|Texas Instruments Incorporated
| MULTI-CHANNEL HIGH SPEED ADC WITH JESD204B INTERFACE
| part#   Digital Voltage Range   Package-type   #pins
| AFE58JD32   1.7V - 1.9V   BGA   289
[IBIS Ver]   4.1
[File name]   afe58jd32.ibs
[File Rev]   1.1
[Date]   9/16/2017
[Source]
| Texas Instruments Incorporated.
| Analog-eLab Design Center, HPA
| 12500 TI Blvd
| Dallas, TX -75243
[Notes]   Revision History:
| Rev 1.0: 7/01/2017
| - Initial version of the model
| - Model generated from simulations in TISPICE
| - C_comp although listed in numerical order of value are
|   obtained from varying PVT conditions. For PVT conditions for
|   each specific value refer the buffer description under
|   respective [Model]. IBIS model user is responsible for using
|   appropriate C_comp to simulate for Signal Integrity.
[Disclaimer]
| This model is designed as an aid for customers of Texas Instruments.
| TI and its licensors and suppliers make no warranties, either expressed
| or implied, with respect to this  model, including the warranties of
| merchantability or fitness for a particular purpose. The model is
| provided solely on an "as is" basis. The entire risk as to its quality
| and performance is with the customer.
[Copyright]
 (C) Copyright 2014 Texas Instruments Incorporated.All rights reserved.
|   Device
[Component]   AFE58JD32
[Manufacturer]   TI
[Package]
|   typ   min   max
R_pkg  1.000E-02   0.800E-02   1.200E-02
L_pkg  1.602E-09   1.280E-09   1.920E-09
C_pkg  0.700E-13   0.560E-13   0.840E-12
[Pin]  signal_name   model_name   R_pin   L_pin   C_pin
A1   INP31   NC   NA   NA   NA
A2   INP29   NC   NA   NA   NA
A3   INP27   NC   NA   NA   NA
A4   INP25   NC   NA   NA   NA
A5   INP23   NC   NA   NA   NA
A6   INP21   NC   NA   NA   NA
A7   INP19   NC   NA   NA   NA
A8   INP17   NC   NA   NA   NA
A9   BIAS_2P5o   NC   NA   NA   NA
A10   INP15   NC   NA   NA   NA
A11   INP13   NC   NA   NA   NA
A12   INP11   NC   NA   NA   NA
A13   INP9   NC   NA   NA   NA
A14   INP7   NC   NA   NA   NA
A15   INP5   NC   NA   NA   NA
A16   INP3   NC   NA   NA   NA
A17   INP1   NC   NA   NA   NA
B1   INM31   NC   NA   NA   NA
B2   INM29   NC   NA   NA   NA
B3   INM27   NC   NA   NA   NA
B4   INM25   NC   NA   NA   NA
B5   INM23   NC   NA   NA   NA
B6   INM21   NC   NA   NA   NA
B7   INM19   NC   NA   NA   NA
B8   INM17   NC   NA   NA   NA
B9   NC   NC   NA   NA   NA
B10   INM15   NC   NA   NA   NA
B11   INM13   NC   NA   NA   NA
B12   INM11   NC   NA   NA   NA
B13   INM9   NC   NA   NA   NA
B14   INM7   NC   NA   NA   NA
B15   INM5   NC   NA   NA   NA
B16   INM3   NC   NA   NA   NA
B17   INM1   NC   NA   NA   NA
C1   INP32   NC   NA   NA   NA
C2   INP30   NC   NA   NA   NA
C3   INP28   NC   NA   NA   NA
C4   INP26   NC   NA   NA   NA
C5   INP24   NC   NA   NA   NA
C6   INP22   NC   NA   NA   NA
C7   INP20   NC   NA   NA   NA
C8   INP18   NC   NA   NA   NA
C9   NC   NC   NA   NA   NA
C10   INP16   NC   NA   NA   NA
C11   INP14   NC   NA   NA   NA
C12   INP12   NC   NA   NA   NA
C13   INP10   NC   NA   NA   NA
C14   INP8   NC   NA   NA   NA
C15   INP6   NC   NA   NA   NA
C16   INP4   NC   NA   NA   NA
C17   INP2   NC   NA   NA   NA
D1   INM32   NC   NA   NA   NA
D2   INM30   NC   NA   NA   NA
D3   INM28   NC   NA   NA   NA
D4   INM26   NC   NA   NA   NA
D5   INM24   NC   NA   NA   NA
D6   INM22   NC   NA   NA   NA
D7   INM20   NC   NA   NA   NA
D8   INM18   NC   NA   NA   NA
D9   BIAS_2P5e   NC   NA   NA   NA
D10   INM16   NC   NA   NA   NA
D11   INM14   NC   NA   NA   NA
D12   INM12   NC   NA   NA   NA
D13   INM10   NC   NA   NA   NA
D14   INM8   NC   NA   NA   NA
D15   INM6   NC   NA   NA   NA
D16   INM4   NC   NA   NA   NA
D17   INM2   NC   NA   NA   NA
E1   AVSS   GND   NA   NA   NA
E2   AVSS   GND   NA   NA   NA
E3   AVSS		GND   NA   NA   NA
E4   LNA_IN_CMe	NC   NA   NA   NA
E5   LNA_IN_CMo   NC   NA   NA   NA
E6   AVDD_3P15   POWER   NA   NA   NA
E7   AVDD_3P15   POWER   NA   NA   NA
E8   NC   NC   NA   NA   NA
E9   NC   NC   NA   NA   NA
E10   AVDD_3P15   POWER   NA   NA   NA
E11   AVDD_3P15   POWER   NA   NA   NA
E12   AVDD_3P15   POWER   NA   NA   NA
E13   SRC_BIASo   NC   NA   NA   NA
E14   SRC_BIASe   NC   NA   NA   NA
E15   AVSS   GND   NA   NA   NA
E16   AVSS   GND   NA   NA   NA
E17   AVSS   GND   NA   NA   NA
F1   CW_OUTP_IP   NC   NA   NA   NA
F2   CW_OUTM_IP   NC   NA   NA   NA
F3   AVSS   GND   NA   NA   NA
F4   NC   NC   NA   NA   NA
F5   NC   NC   NA   NA   NA
F6   AVDD_1P9   POWER   NA   NA   NA
F7   AVDD_1P9   POWER   NA   NA   NA
F8   AVSS   GND   NA   NA   NA
F9   AVSS   GND   NA   NA   NA
F10   AVSS   GND   NA   NA   NA
F11   AVDD_1P9   POWER   NA   NA   NA
F12   AVDD_1P9   POWER   NA   NA   NA
F13   NC   NC   NA   NA   NA
F14   NC   NC   NA   NA   NA
F15   AVSS   GND   NA   NA   NA
F16   CLKP_16X   CLK_INPUT   NA   NA   NA
F17   CLKM_16X   CLK_INPUT   NA   NA   NA
G1   CW_OUTP_QP   NC   NA   NA   NA
G2   CW_OUTM_QP   NC   NA   NA   NA
G3   AVSS   GND   NA   NA   NA
G4   BAND_GAPe   NC   NA   NA   NA
G5   BAND_GAPo   NC   NA   NA   NA
G6   AVDD_1P9   POWER   NA   NA   NA
G7   AVDD_1P9   POWER   NA   NA   NA
G8   AVSS   GND   NA   NA   NA
G9   AVSS   GND   NA   NA   NA
G10   AVSS   GND   NA   NA   NA
G11   AVDD_1P9   POWER   NA   NA   NA
G12   AVDD_1P9   POWER   NA   NA   NA
G13   NC   NC   NA   NA   NA
G14   NC   NC   NA   NA   NA
G15   AVSS   GND   NA   NA   NA
G16   AVSS   GND   NA   NA   NA
G17   AVSS   GND   NA   NA   NA
H1   AVSS   GND   NA   NA   NA
H2   AVSS   GND   NA   NA   NA
H3   AVSS   GND   NA   NA   NA
H4   TGC_SLOPE   NC   NA   NA   NA
H5   TGC_PROF2   NC   NA   NA   NA
H6   AVDD_1P9   POWER   NA   NA   NA
H7   AVDD_1P9   POWER   NA   NA   NA
H8   AVSS   GND   NA   NA   NA
H9   AVSS   GND   NA   NA   NA
H10   AVSS   GND   NA   NA   NA
H11   AVDD_1P9   POWER   NA   NA   NA
H12   AVDD_1P9   POWER   NA   NA   NA
H13   AVDD_1P9   POWER   NA   NA   NA
H14   TR_EN2   NC   NA   NA   NA
H15   TR_EN3   NC   NA   NA   NA
H16   CLKM_1X   CLK_INPUT   NA   NA   NA
H17   CLKP_1X   CLK_INPUT   NA   NA   NA
J1   ADC_CLKP   CLK_INPUT   NA   NA   NA
J2   ADC_CLKM   CLK_INPUT   NA   NA   NA
J3   AVSS   GND   NA   NA   NA
J4   TGC_UP_DN   NC   NA   NA   NA
J5   TGC_PROF1   NC   NA   NA   NA
J6   AVDD_1P9   POWER   NA   NA   NA
J7   AVDD_1P9   POWER   NA   NA   NA
J8   AVSS   GND   NA   NA   NA
J9   AVSS   GND   NA   NA   NA
J10   AVSS   GND   NA   NA   NA
J11   AVDD_1P9   POWER   NA   NA   NA
J12   AVDD_1P9   POWER   NA   NA   NA
J13   NC   NC   NA   NA   NA
J14   TR_EN1   NC   NA   NA   NA
J15   TR_EN4   NC   NA   NA   NA
J16   SDOUT   SDOUT   NA   NA   NA
J17   SCLK   SCLK_INPUT   NA   NA   NA
K1   AVSS   GND   NA   NA   NA
K2   AVSS   GND   NA   NA   NA
K3   AVSS   GND   NA   NA   NA
K4   NC   NC   NA   NA   NA
K5   NC   NC   NA   NA   NA
K6   AVDD_1P8   POWER   NA   NA   NA
K7   AVDD_1P8   POWER   NA   NA   NA
K8   AVSS   GND   NA   NA   NA
K9   AVSS   GND   NA   NA   NA
K10   AVSS   GND   NA   NA   NA
K11   AVDD_1P8   POWER   NA   NA   NA
K12   AVDD_1P8   POWER   NA   NA   NA
K13   NC   NC   NA   NA   NA
K14   NC   NC   NA   NA   NA
K15   SENo   SEN   NA   NA   NA
K16   SPI_DIG_EN   SEN   NA   NA   NA
K17   SENe   SEN   NA   NA   NA
L1   SYNCP_SERDES   SYNC_INPUT   NA   NA   NA
L2   SYNCM_SERDES   SYNC_INPUT   NA   NA   NA
L3   DVDD_1P2   POWER   NA   NA   NA
L4   NC   NC   NA   NA   NA
L5   NC   NC   NA   NA   NA
L6   AVDD_1P8   POWER   NA   NA   NA
L7   AVDD_1P8   POWER   NA   NA   NA
L8   AVSS   GND   NA   NA   NA
L9   AVSS   GND   NA   NA   NA
L10   AVSS   GND   NA   NA   NA
L11   AVDD_1P8   POWER   NA   NA   NA
L12   AVDD_1P8   POWER   NA   NA   NA
L13   NC   NC   NA   NA   NA
L14   NC   NC   NA   NA   NA
L15   NC   NC   NA   NA   NA
L16   SDIN   SCLK_INPUT   NA   NA   NA
L17   RESET   SCLK_INPUT   NA   NA   NA
M1   SYSREFP_SERDES   SYNC_INPUT   NA   NA   NA
M2   SYSREFM_SERDES   SYNC_INPUT   NA   NA   NA
M3   DVSS   GND   NA   NA   NA
M4   DVDD_1P2   POWER   NA   NA   NA
M5   DVDD_1P2   POWER   NA   NA   NA
M6   DVDD_1P2   POWER   NA   NA   NA
M7   DVSS   GND   NA   NA   NA
M8   DVSS   GND   NA   NA   NA
M9   DVSS   GND   NA   NA   NA
M10   DVSS   GND   NA   NA   NA
M11   DVSS   GND   NA   NA   NA
M12   DVDD_1P2   POWER   NA   NA   NA
M13   DVDD_1P2   POWER   NA   NA   NA
M14   DVDD_1P2   POWER   NA   NA   NA
M15   TX_TRIG   SCLK_INPUT   NA   NA   NA
M16   PDN_GBL   SCLK_INPUT   NA   NA   NA
M17   PDN_FAST   SCLK_INPUT   NA   NA   NA
N1   CML5_OUTP   CML_OUT   NA   NA   NA
N2   DVDD_1P2   POWER   NA   NA   NA
N3   DVDD_1P2   POWER   NA   NA   NA
N4   DVDD_1P2   POWER   NA   NA   NA
N5   DVDD_1P2   POWER   NA   NA   NA
N6   DVDD_1P2   POWER   NA   NA   NA
N7   DVSS   GND   NA   NA   NA
N8   DVSS   GND   NA   NA   NA
N9   DVSS   GND   NA   NA   NA
N10   DVSS   GND   NA   NA   NA
N11   DVSS   GND   NA   NA   NA
N12   DVDD_1P2   POWER   NA   NA   NA
N13   DVDD_1P2   POWER   NA   NA   NA
N14   DVDD_1P2   POWER   NA   NA   NA
N15   DVDD_1P2   POWER   NA   NA   NA
N16   DVDD_1P2   POWER   NA   NA   NA
N17   CML1_OUTP   CML_OUT   NA   NA   NA
P1   CML5_OUTM   CML_OUT   NA   NA   NA
P2   DVDD_1P2   POWER   NA   NA   NA
P3   DVDD_1P2   POWER   NA   NA   NA
P4   DVDD_1P8   POWER   NA   NA   NA
P5   DVDD_1P8   POWER   NA   NA   NA
P6   DVDD_1P8   POWER   NA   NA   NA
P7   DVDD_1P8   POWER   NA   NA   NA
P8   DVSS   GND   NA   NA   NA
P9   DVSS   GND   NA   NA   NA
P10   DVSS   GND   NA   NA   NA
P11   DVDD_1P8   POWER   NA   NA   NA
P12   DVDD_1P8   POWER   NA   NA   NA
P13   DVDD_1P8   POWER   NA   NA   NA
P14   DVDD_1P8   POWER   NA   NA   NA
P15   DVDD_1P2   POWER   NA   NA   NA
P16   DVDD_1P2   POWER   NA   NA   NA
P17   CML1_OUTM   CML_OUT   NA   NA   NA
R1   CML6_OUTP   CML_OUT   NA   NA   NA
R2   DOUTP16   LVDS_OUT   NA   NA   NA
R3   DOUTP15   LVDS_OUT   NA   NA   NA
R4   DOUTP14   LVDS_OUT   NA   NA   NA
R5   NC   NC   NA   NA   NA
R6   DOUTM11   LVDS_OUT   NA   NA   NA
R7   DOUTP11   LVDS_OUT   NA   NA   NA
R8   FCLKM   LVDS_OUT   NA   NA   NA
R9   NC   NC   NA   NA   NA
R10   FCLKP   LVDS_OUT   NA   NA   NA
R11   DOUTM6   LVDS_OUT   NA   NA   NA
R12   DOUTP6   LVDS_OUT   NA   NA   NA
R13   NC   NC   NA   NA   NA
R14   DOUTP3   LVDS_OUT   NA   NA   NA
R15   DOUTP2   LVDS_OUT   NA   NA   NA
R16   DOUTP1   LVDS_OUT   NA   NA   NA
R17   CML2_OUTP   CML_OUT   NA   NA   NA
T1   CML6_OUTM   CML_OUT   NA   NA   NA
T2   DOUTM16   LVDS_OUT   NA   NA   NA
T3   DOUTM15   LVDS_OUT   NA   NA   NA
T4   DOUTM14   LVDS_OUT   NA   NA   NA
T5   DOUTP13   LVDS_OUT   NA   NA   NA
T6   DOUTP12   LVDS_OUT   NA   NA   NA
T7   DOUTP10   LVDS_OUT   NA   NA   NA
T8   DOUTP9   LVDS_OUT   NA   NA   NA
T9   DCLKP   LVDS_OUT   NA   NA   NA
T10   DOUTP8   LVDS_OUT   NA   NA   NA
T11   DOUTP7   LVDS_OUT   NA   NA   NA
T12   DOUTP5   LVDS_OUT   NA   NA   NA
T13   DOUTP4   LVDS_OUT   NA   NA   NA
T14   DOUTM3   LVDS_OUT   NA   NA   NA
T15   DOUTM2   LVDS_OUT   NA   NA   NA
T16   DOUTM1   LVDS_OUT   NA   NA   NA
T17   CML2_OUTM   CML_OUT   NA   NA   NA
U1   CML7_OUTP   CML_OUT   NA   NA   NA
U2   CML7_OUTM   CML_OUT   NA   NA   NA
U3   CML8_OUTP   CML_OUT   NA   NA   NA
U4   CML8_OUTM   CML_OUT   NA   NA   NA
U5   DOUTM13   LVDS_OUT   NA   NA   NA
U6   DOUTM12   LVDS_OUT   NA   NA   NA
U7   DOUTM10   LVDS_OUT   NA   NA   NA
U8   DOUTM9   LVDS_OUT   NA   NA   NA
U9   DCLKM   LVDS_OUT   NA   NA   NA
U10   DOUTM8   LVDS_OUT   NA   NA   NA
U11   DOUTM7   LVDS_OUT   NA   NA   NA
U12   DOUTM5   LVDS_OUT   NA   NA   NA
U13   DOUTM4   LVDS_OUT   NA   NA   NA
U14   CML4_OUTM   CML_OUT   NA   NA   NA
U15   CML4_OUTP   CML_OUT   NA   NA   NA
U16   CML3_OUTM   CML_OUT   NA   NA   NA
U17   CML3_OUTP   CML_OUT   NA   NA   NA
[Diff Pin]  inv_pin  vdiff  tdelay_typ tdelay_min tdelay_max
J1   J2   NA   NA   NA   NA
T9   U9   NA   NA   NA   NA
H17   H16   NA   NA   NA   NA
F16   F17   NA   NA   NA   NA
N1   P1   NA   NA   NA   NA
N17  P17   NA   NA   NA   NA
R17  T17   NA   NA   NA   NA
U17 U16   NA   NA   NA   NA
U15   U14   NA   NA   NA   NA
R1   T1   NA   NA   NA   NA
U1   U2   NA   NA   NA   NA
U3   U4   NA   NA   NA   NA
R16  T16   NA   NA   NA   NA
R15  T15   NA   NA   NA   NA
R14  T14   NA   NA   NA   NA
T13  U13   NA   NA   NA   NA
T12  U12   NA   NA   NA   NA
R12  R11   NA   NA   NA   NA
T11  U11   NA   NA   NA   NA
T10  U10   NA   NA   NA   NA
T8   U8   NA   NA   NA   NA
T7  U7   NA   NA   NA   NA
R7  R6   NA   NA   NA   NA
T6  U6   NA   NA   NA   NA
T5  U5   NA   NA   NA   NA
R4  T4   NA   NA   NA   NA
R3  T3   NA   NA   NA   NA
R2  T2   NA   NA   NA   NA
L1  L2   NA   NA   NA   NA
M1  M2   NA   NA   NA   NA
R10  R8   NA   NA   NA   NA
|   Model Selectors
[Model Selector]  SDOUT
SDOUT_OUTPUT0  SDOUT buffer with CMOS process
SDOUT_OUTPUT1 SDOUT buffer with other process
[Model Selector]  SCLK_INPUT
SCLK_INPUT0  SCLK buffer with CMOS process
SCLK_INPUT1 SCLK buffer with other process
[Model Selector]  SEN
SEN_INPUT0  SEN buffer with CMOS process
SEN_INPUT1 SEN buffer with other process
| Models and submodels in the file (10): SCLK_INPUT0 (Input), SCLK_INPUT1 (Input), CML_OUT (Output), LVDS_OUT (Output), SDOUT_OUTPUT0 (Output), SDOUT_OUTPUT1 (Output), SYNC_INPUT (Input), SEN_INPUT0 (Input), SEN_INPUT1 (Input), CLK_INPUT (Input)
